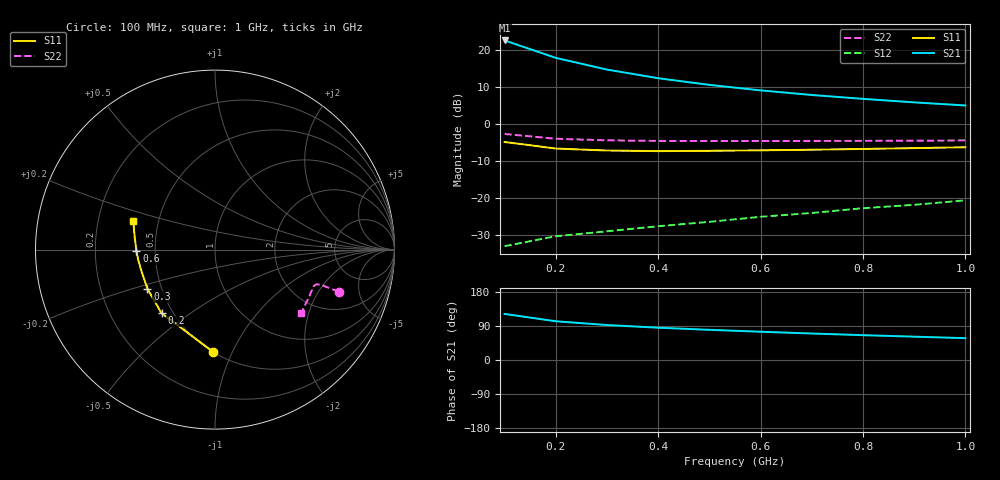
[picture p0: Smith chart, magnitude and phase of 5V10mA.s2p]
#  HZ  S  MA  R  50.0000
! Device:15GN03CA
! "! Bias:VCE=5V, IC=10mA  "
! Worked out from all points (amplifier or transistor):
!   10 points, 100 MHz to 1 GHz, reference 50 ohm
!   highest |S21| = 22.6 dB at 100 MHz (marker M1)
!   |S21| within 3 dB of that: start of sweep to 163.6 MHz
!   unconditionally stable (mu >= 1): 207.5 MHz to end of sweep
!   at 200 MHz: K = 0.98, MSG = 24.2 dB, |S12| = -30.5 dB
!   at 600 MHz: K = 1.53, MAG = 12.8 dB, |S12| = -25.2 dB
!   at 1 GHz: K = 1.32, MAG = 9.5 dB, |S12| = -20.7 dB
!   S11 on the Smith chart (normalised r, x): 100 MHz: 0.50, -0.84; 200 MHz: 0.43, -0.39; 300 MHz: 0.42, -0.22; 600 MHz: 0.39, -0.01; 1 GHz: 0.36, +0.15
1e8  0.568 -91.3  13.49 121.5  0.022 51.2  0.729 -18.8
2e8  0.463 -130.0  7.837 102.2  0.03 50.0  0.628 -18.4
3e8  0.435 -149.9  5.435 92.3  0.035 56.5  0.598 -18.8
4e8  0.427 -162.7  4.153 85.2  0.041 60.0  0.587 -20.2
5e8  0.431 -171.8  3.374 79.6  0.047 67.1  0.586 -22.4
6e8  0.438 -179.1  2.842 74.6  0.055 70.4  0.585 -24.6
7e8  0.446 174.7  2.46 69.9  0.062 74.5  0.587 -27.4
8e8  0.457 169.2  2.181 65.5  0.072 78.2  0.588 -30.3
9e8  0.469 164.7  1.954 61.6  0.08 80.5  0.592 -33.5
1e9  0.482 160.6  1.775 57.6  0.092 82.6  0.596 -36.4
